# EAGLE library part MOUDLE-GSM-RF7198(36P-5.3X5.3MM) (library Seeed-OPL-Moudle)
317010002
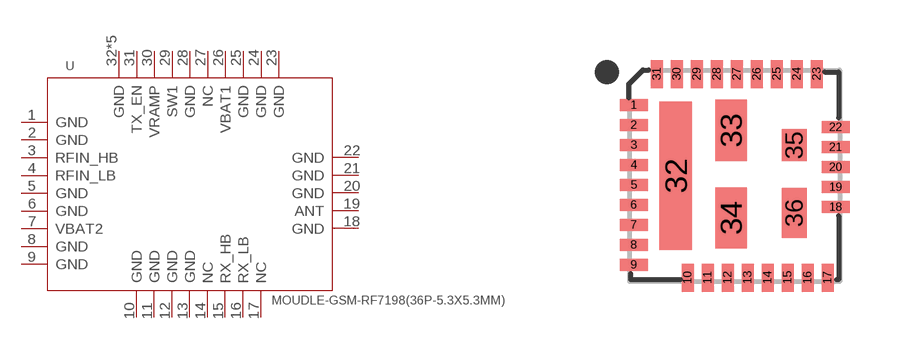
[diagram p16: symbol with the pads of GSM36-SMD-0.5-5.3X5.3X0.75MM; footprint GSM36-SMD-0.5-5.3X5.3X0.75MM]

Designator prefix U

## MOUDLE-GSM-RF7198(36P-5.3X5.3MM) (MPN: RF7198; VALUE: RF7198)  [GSM36-SMD-0.5-5.3X5.3X0.75MM]
1  GND
2  GND
3  RFIN_HB
4  RFIN_LB  pas
5  GND  pas
6  GND  pas
7  VBAT2  pas
8  GND  pas
9  GND  pas
10  GND  pas
11  GND  pas
12  GND  pas
13  GND  pas
14  NC  pas
15  RX_HB  pas
16  RX_LB  pas
17  NC  pas
18  GND  pas
19  ANT  pas
20  GND  pas
21  GND  pas
22  GND  pas
23  GND  pas
24  GND  pas
25  GND  pas
26  VBAT1  pas
27  NC  pas
28  GND  pas
29  SW1  pas
30  VRAMP  pas
31  TX_EN  pas
32  GND  pas
33  GND  pas
34  GND  pas
35  GND  pas
36  GND  pas

## Footprint GSM36-SMD-0.5-5.3X5.3X0.75MM (pad centres in mm)
smd 0.7 x 0.3: 1 -2.525,1.77; 2 -2.525,1.27; 3 -2.525,0.77; 4 -2.525,0.27; 5 -2.525,-0.23; 6 -2.525,-0.73; 7 -2.525,-1.23; 8 -2.525,-1.73; 9 -2.525,-2.23; 18 2.525,-0.785; 19 2.525,-0.285; 20 2.525,0.215; 21 2.525,0.715; 22 2.525,1.215
smd 0.3 x 0.7: 10 -1.175,-2.55; 11 -0.675,-2.55; 12 -0.175,-2.55; 13 0.325,-2.55; 14 0.825,-2.55; 15 1.325,-2.55; 16 1.825,-2.55; 17 2.325,-2.55; 23 2.055,2.55; 24 1.555,2.55; 25 1.055,2.55; 26 0.555,2.55; 27 0.055,2.55; 28 -0.445,2.55; 29 -0.945,2.55; 30 -1.445,2.55; 31 -1.945,2.55
smd 0.805 x 3.715: 32 -1.473,0
smd 0.785 x 1.535: 33 -0.083,1.133; 34 -0.083,-1.055
smd 0.635 x 0.8: 35 1.493,0.765
smd 0.635 x 1.245: 36 1.493,-0.933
